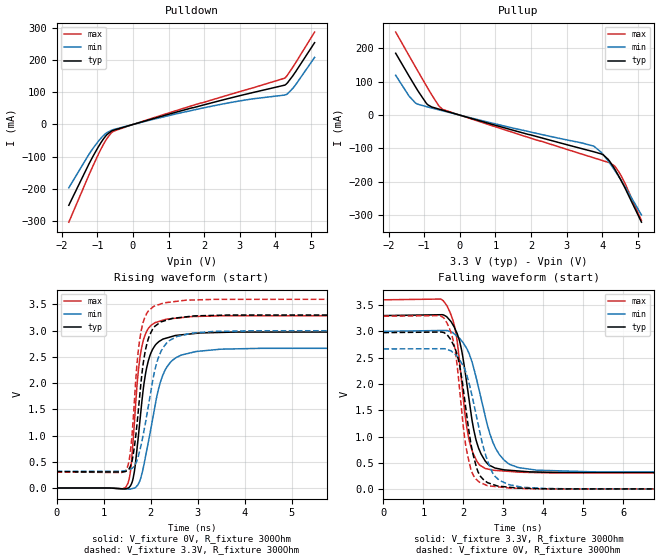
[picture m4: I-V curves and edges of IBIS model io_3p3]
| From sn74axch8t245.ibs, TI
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|   io_3p3 Model
[Model]   io_3p3
Model_type   I/O
Polarity   Non-Inverting
Enable   Active-High
Vinl = 0.8
Vinh = 2.0
Vmeas = 1.65
Vref = 0
Cref = 2pF
Rref = 100000
|   typ   min   max
C_comp   2.5215E-12   1.93928E-12   2.79024E-12
| Where Nom  PVT is Nominal Process, 3.3V, 27C
|   Fast PVT is Strong Process,  3.6V, -40C
|   Slow PVT is Weak Process,   3.0V, 130C
[Voltage Range]   3.3   3   3.6
|Junction Temperature
[Temperature Range]   27   130   -40
[Pullup Reference]   3.3   3   3.6
[Pulldown Reference]   -0   0   0
[Power Clamp Reference]   3.3   3   3.6
[GND Clamp Reference]   0   0   0
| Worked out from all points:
|   slope of the pulldown table from 0 to 0.495 V, typ, clamps not added: 31.4 ohm
|   slope of the pullup table from 0 to 0.495 V, typ, clamps not added: 32.7 ohm
|   falling waveform, V_fixture 3.3V, R_fixture 300Ohm: 20-80 % time 387ps typ, 563ps min, 317ps max; typ from 3.3 V to 0.311 V
|   rising waveform, V_fixture 0V, R_fixture 300Ohm: 20-80 % time 247ps typ, 375ps min, 194ps max; typ from 0 V to 2.98 V
|   rising waveform, V_fixture 3.3V, R_fixture 300Ohm: 20-80 % time 236ps typ, 351ps min, 189ps max; typ from 0.311 V to 3.3 V
|   falling waveform, V_fixture 0V, R_fixture 300Ohm: 20-80 % time 366ps typ, 510ps min, 306ps max; typ from 2.98 V to 0 V
[Pulldown]
|   Voltage   I(typ)   I(min)   I(max)
-1.8V     -250.7mA   -196.3mA   -303.2mA
-1.241V   -123.8mA   -93.74mA   -158.3mA
-972mV    -69.58mA   -52.19mA   -93.01mA
-737.4mV  -32.43mA   -25.88mA   -44.75mA
-592.5mV  -20.1mA    -17.51mA   -24.67mA
145.8mV   4.68mA     4.106mA    5.242mA
2.271V    68.91mA    58.08mA    78.04mA
3.237V    95.62mA    77.35mA    109.5mA
4.265V    122.2mA    91.32mA    143.8mA
4.341V    129.5mA    95.35mA    153.7mA
4.52V     156mA      116.5mA    183.3mA
5.1V      253.7mA    208mA      286.6mA
[Pullup]
|   Voltage   I(typ)   I(min)   I(max)
-1.8V     185.6mA    119.5mA    249.1mA
-1.427V   117.5mA    57.51mA    178.8mA
-1.241V   84.3mA     35.92mA    143.9mA
-944.4mV  36.23mA    25.73mA    89.06mA
-592.5mV  18.28mA    16.01mA    28.28mA
-482.1mV  14.86mA    13mA       17.29mA
3.761V    -109.8mA   -92.92mA   -128.1mA
4.03V     -119.5mA   -118.7mA   -137mA
4.168V    -133.1mA   -137.7mA   -141.7mA
4.369V    -165.2mA   -168.7mA   -155.5mA
4.638V    -218.5mA   -214.6mA   -204.3mA
5.1V      -321.1mA   -299.4mA   -316.2mA
[Ramp]
R_load = 300
|   typ   min   max
dV/dt_r   1.7857/2.46318e-10   1.59971/3.74481e-10   1.97252/1.92611e-10
dV/dt_f   1.79321/3.86651e-10   1.60856/5.60378e-10   1.97637/3.16088e-10
[Falling Waveform]
V_fixture = 3.3V
V_fixture_min = 3V
V_fixture_max = 3.6V
R_fixture = 300Ohm
C_fixture = 0F
|   Time   V(typ)   V(min)   V(max)
0s        3.3V       3V         3.6V
1.581ns   3.28V      3.016V     3.497V
1.787ns   3.055V     2.943V     3.073V
1.904ns   2.819V     2.869V     2.432V
2.192ns   1.441V     2.474V     795.1mV
2.38ns    783.1mV    1.933V     486.6mV
2.757ns   414.6mV    859.8mV    359.5mV
3.382ns   345.6mV    410.1mV    323.8mV
5.461ns   316.3mV    324.4mV    310.4mV
30ns      311.3mV    319.1mV    306mV
[Rising Waveform]
V_fixture = 0V
V_fixture_min = 0V
V_fixture_max = 0V
R_fixture = 300Ohm
C_fixture = 0F
|   Time   V(typ)   V(min)   V(max)
0s        54.99nV    84.96nV    -90.27nV
1.469ns   -13.86mV   -17.68mV   10.4mV
1.562ns   32.37mV    -22.15mV   263.6mV
1.65ns    295.4mV    -1.784mV   1.196V
1.739ns   992.5mV    78.68mV    2.242V
1.842ns   1.88V      380.9mV    2.809V
2.002ns   2.566V     1.121V     3.092V
2.334ns   2.856V     2.29V      3.217V
4.365ns   2.972V     2.662V     3.283V
30ns      2.976V     2.666V     3.288V
[Rising Waveform]
V_fixture = 3.3V
V_fixture_min = 3V
V_fixture_max = 3.6V
R_fixture = 300Ohm
C_fixture = 0F
|   Time   V(typ)   V(min)   V(max)
0s        311.3mV    319.1mV    306mV
1.461ns   312.7mV    330.6mV    322.4mV
1.552ns   384.6mV    354.7mV    583.2mV
1.624ns   611.3mV    390.2mV    1.256V
1.732ns   1.421V     586.8mV    2.575V
1.827ns   2.278V     953.2mV    3.114V
1.983ns   2.923V     1.73V      3.397V
2.286ns   3.183V     2.702V     3.528V
4.175ns   3.296V     2.996V     3.595V
30ns      3.3V       3V         3.6V
[Falling Waveform]
|Gnd
V_fixture = 0V
V_fixture_min = 0V
V_fixture_max = 0V
R_fixture = 300Ohm
C_fixture = 0F
|   Time   V(typ)   V(min)   V(max)
0s        2.976V     2.666V     3.288V
1.529ns   2.97V      2.67V      3.237V
1.732ns   2.774V     2.604V     2.874V
1.872ns   2.477V     2.5V       2.157V
2.027ns   1.74V      2.297V     1.011V
2.175ns   931.2mV    1.912V     414.7mV
2.61ns    122.4mV    532.6mV    64.78mV
2.912ns   55.75mV    163.5mV    40.61mV
3.957ns   9.367mV    14.76mV    4.877mV
30ns      -89.6nV    327.2nV    24.16nV
